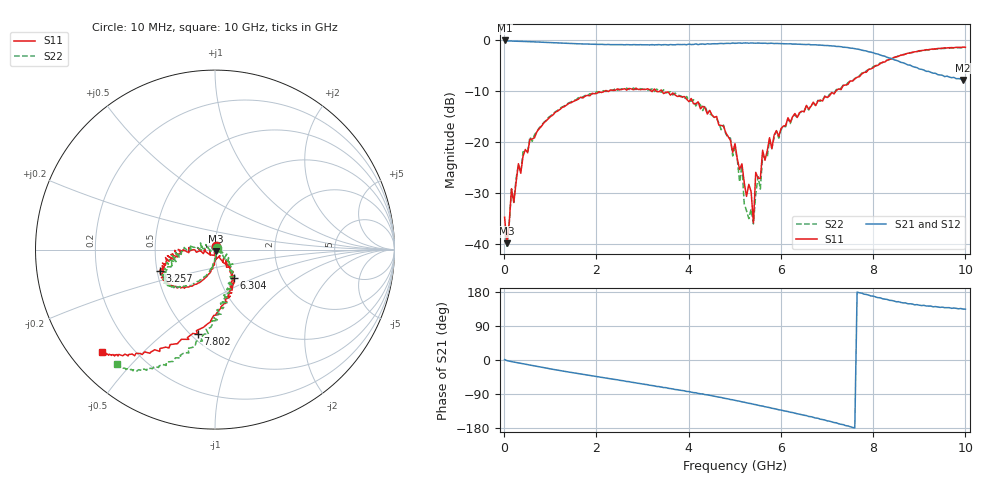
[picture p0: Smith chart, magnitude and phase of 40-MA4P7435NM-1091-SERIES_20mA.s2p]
!Agilent Technologies,E8364C,MY48140145,A.09.42.15
!Agilent E8364C: A.09.42.15
!Date: Wednesday, December 02, 2020 13:41:24
!Correction: S11(Full 2 Port(1,2))
!S21(Full 2 Port(1,2))
!S12(Full 2 Port(1,2))
!S22(Full 2 Port(1,2))
!S2P File: Measurements: S11, S21, S12, S22:
# Hz S  dB  R 50
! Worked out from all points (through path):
!   201 points, 10 MHz to 10 GHz, reference 50 ohm
!   highest |S21| = -0.11 dB at 10 MHz (marker M1); lowest = -7.9 dB at 9.95 GHz (marker M2)
!   group delay of S21, straight-line fit = 66.1 ps
!   lowest |S11| = -39.8 dB at 59.95 MHz (marker M3), VSWR 1.02, Z = 50.5 - j0.878 ohm
!   |S11| at or under -10 dB: start of sweep to 2.187 GHz; 3.296 GHz to 3.377 GHz (80.98 MHz wide, 2.43 % of centre); 3.421 GHz to 7.194 GHz (3.772 GHz wide, 71.1 % of centre)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
!   |S22| runs from -40.4 to -1.5 dB; largest |S21 - S12| = 0.025
!   S11 on the Smith chart (normalised r, x): 10 MHz: 1.01, +0.04; 3.257 GHz: 0.52, -0.14; 6.304 GHz: 1.17, -0.38; 7.802 GHz: 0.54, -0.66; 10 GHz: 0.09, -0.38
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1e7  -34.68 69.7  -0.11 1.0  -0.07 -0.5  -36.47 36.6
5.995e7  -39.82 -58.3  -0.19 -1.5  -0.19 -1.6  -40.36 -70.8
1.5985e8  -29.12 -79.8  -0.22 -4.2  -0.22 -4.2  -29.20 -78.7
5.5945e8  -19.48 -98.8  -0.37 -13.6  -0.36 -13.6  -18.99 -98.6
1.7083e9  -11.35 -129.5  -0.77 -38.0  -0.76 -37.7  -11.14 -132.5
3.25675e9  -9.59 -158.9  -0.98 -68.2  -0.94 -68.8  -10.10 -150.5
3.35665e9  -10.14 -160.2  -0.92 -70.1  -0.95 -70.6  -9.98 -150.8
5.005e9  -20.31 174.3  -0.67 -106.5  -0.62 -106.6  -21.01 155.4
5.1049e9  -25.35 178.0  -0.59 -108.8  -0.60 -109.1  -27.80 167.7
5.15485e9  -24.25 -175.5  -0.65 -110.4  -0.62 -110.3  -24.58 151.8
5.2048e9  -27.90 -133.6  -0.59 -111.4  -0.62 -111.2  -32.03 -157.5
5.35465e9  -29.69 -85.7  -0.60 -115.1  -0.61 -115.2  -33.11 -48.6
5.4046e9  -35.83 -104.3  -0.62 -116.8  -0.60 -116.9  -36.02 42.5
5.45455e9  -25.92 -77.5  -0.65 -117.8  -0.63 -117.7  -30.18 -50.0
5.55445e9  -27.13 -62.7  -0.65 -120.8  -0.64 -120.8  -29.20 -19.6
5.6044e9  -21.60 -57.4  -0.66 -121.6  -0.66 -121.6  -22.65 -43.9
6.3037e9  -14.40 -56.5  -0.81 -140.3  -0.81 -140.3  -14.63 -53.1
6.7033e9  -12.18 -67.3  -0.96 -151.4  -0.95 -151.4  -12.44 -65.9
7.8022e9  -6.36 -101.6  -2.09 173.9  -2.04 174.5  -6.49 -97.2
8.35165e9  -3.80 -118.5  -3.54 157.5  -3.46 158.4  -3.85 -110.1
9.95005e9  -1.41 -137.4  -7.86 134.4  -7.77 135.4  -1.52 -130.1
1e10  -1.43 -137.9  -7.79 134.1  -7.80 134.0  -1.51 -130.5
